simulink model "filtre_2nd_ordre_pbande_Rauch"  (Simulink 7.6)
settings: Solver=ode45  StartTime=0.0  StopTime=10.0  RelTol=1e-3
libraries: fl_lib x8, elec_lib x3, nesl_utility x3

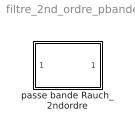
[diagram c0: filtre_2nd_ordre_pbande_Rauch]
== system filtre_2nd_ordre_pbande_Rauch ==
  passe bande Rauch_2ndordre : Subsystem

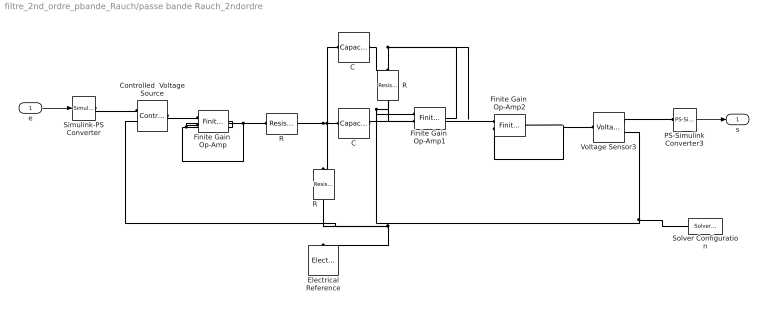
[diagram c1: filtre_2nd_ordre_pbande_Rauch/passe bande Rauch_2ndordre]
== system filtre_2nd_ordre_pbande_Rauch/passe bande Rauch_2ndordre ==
  e : Inport
  C : fl_lib/Electrical/Electrical Elements/Capacitor  DialogController=NetworkEngine.DynNeDlgSource  SystemSampleTime=-1  c=1e-6 F  v0=0 V  r=1e-6 Ohm  g=0 1/Ohm  i_Log=off  v_Log=off  vc_Log=off  LocalVarNames=|i|v|vc  LocalVarDescs=|i|v|Internal variable for voltage across capacitor term  LocalVarLogging=[0 0 0]
  "C " : fl_lib/Electrical/Electrical Elements/Capacitor  DialogController=NetworkEngine.DynNeDlgSource  SystemSampleTime=-1  c=1e-6 F  v0=0 V  r=1e-6 Ohm  g=0 1/Ohm  i_Log=off  v_Log=off  vc_Log=off  LocalVarNames=|i|v|vc  LocalVarDescs=|i|v|Internal variable for voltage across capacitor term  LocalVarLogging=[0 0 0]
  Controlled  Voltage Source : fl_lib/Electrical/Electrical Sources/Controlled Voltage Source  DialogController=NetworkEngine.DynNeDlgSource  SystemSampleTime=-1  i_Log=off  v_Log=off  LocalVarNames=|i|v  LocalVarDescs=|i|v  LocalVarLogging=[0 0]
  Electrical Reference : fl_lib/Electrical/Electrical Elements/Electrical Reference  DialogController=NetworkEngine.DynNeDlgSource  SystemSampleTime=-1  i_Log=off  LocalVarNames=|i  LocalVarDescs=|i  LocalVarLogging=0
  Finite Gain  Op-Amp : elec_lib/Integrated Circuits/Finite Gain Op-Amp  DialogController=NetworkEngine.DynNeDlgSource  SystemSampleTime=-1  A=1000  Rin=1e+6 Ohm  Rout=100 Ohm  Vmin=-15 V  Vmax=15 V  LocalVarLogging=[]
  Finite Gain  Op-Amp1 : elec_lib/Integrated Circuits/Finite Gain Op-Amp  DialogController=NetworkEngine.DynNeDlgSource  SystemSampleTime=-1  A=1000  Rin=1e+6 Ohm  Rout=100 Ohm  Vmin=-15 V  Vmax=15 V  LocalVarLogging=[]
  Finite Gain  Op-Amp2 : elec_lib/Integrated Circuits/Finite Gain Op-Amp  DialogController=NetworkEngine.DynNeDlgSource  SystemSampleTime=-1  A=1000  Rin=1e+6 Ohm  Rout=100 Ohm  Vmin=-15 V  Vmax=15 V  LocalVarLogging=[]
  PS-Simulink Converter3 : nesl_utility/PS-Simulink Converter  DialogController=NetworkEngine.DynNeUtilDlgSource  SystemSampleTime=-1  PhysicalDomain=network_engine_domain  LeftPortType=input  RightPortType=output  SubClassName=ps_output  Unit=1  AffineConversion=off
  R : fl_lib/Electrical/Electrical Elements/Resistor  DialogController=NetworkEngine.DynNeDlgSource  SystemSampleTime=-1  R=1 Ohm  i_Log=off  v_Log=off  LocalVarNames=|i|v  LocalVarDescs=|i|v  LocalVarLogging=[0 0]
  "R " : fl_lib/Electrical/Electrical Elements/Resistor  DialogController=NetworkEngine.DynNeDlgSource  SystemSampleTime=-1  R=1 Ohm  i_Log=off  v_Log=off  LocalVarNames=|i|v  LocalVarDescs=|i|v  LocalVarLogging=[0 0]
  "R   " : fl_lib/Electrical/Electrical Elements/Resistor  DialogController=NetworkEngine.DynNeDlgSource  SystemSampleTime=-1  R=1 Ohm  i_Log=off  v_Log=off  LocalVarNames=|i|v  LocalVarDescs=|i|v  LocalVarLogging=[0 0]
  Simulink-PS Converter : nesl_utility/Simulink-PS Converter  DialogController=NetworkEngine.DynNeUtilDlgSource  SystemSampleTime=-1  PhysicalDomain=network_engine_domain  LeftPortType=input  RightPortType=output  SubClassName=ps_input  Unit=1  AffineConversion=off  InputFilterTimeConstant=.001  UdotUserProvided=0
  Solver Configuration : nesl_utility/Solver Configuration  DialogController=NetworkEngine.DynNeUtilDlgSource  SystemSampleTime=-1  PhysicalDomain=network_engine_domain  LeftPortType=input  RightPortType=generic  SubClassName=solver  Accelerate=off  Profile=off  ResidualTolerance=1e-9  MaxNonlinIter=12  MaxModeIter=2  DoFixedCost=off  UseLocalSampling=off  DoDC=off  LinearAlgebra=Sparse  LocalSolverSampleTime=.001  LocalSolverChoice=NE_BACKWARD_EULER_ADVANCER  UseLocalSolver=off
  Voltage Sensor3 : fl_lib/Electrical/Electrical Sensors/Voltage Sensor  DialogController=NetworkEngine.DynNeDlgSource  SystemSampleTime=-1  i1_Log=off  v1_Log=off  LocalVarNames=|i1|v1  LocalVarDescs=|i1|v1  LocalVarLogging=[]
  s : Outport
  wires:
  PS-Simulink Converter3/1 -> s/1
  e/1 -> Simulink-PS Converter/1
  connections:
  C/LConn1 -- R/RConn1 -- "R "/LConn1 -- "C "/LConn1
  C/RConn1 -- Finite Gain  Op-Amp1/LConn2
  "C "/RConn1 -- "R   "/LConn1 -- Finite Gain  Op-Amp1/RConn1 -- Finite Gain  Op-Amp2/LConn1
  Voltage Sensor3/RConn2 -- "R "/RConn1 -- Electrical Reference/LConn1 -- Controlled  Voltage Source/RConn2 -- Finite Gain  Op-Amp1/LConn1 -- "R   "/RConn1 -- Solver Configuration/RConn1
  Finite Gain  Op-Amp/LConn2 -- Finite Gain  Op-Amp/RConn1 -- R/LConn1
  Finite Gain  Op-Amp2/LConn2 -- Finite Gain  Op-Amp2/RConn1 -- Voltage Sensor3/LConn1
  Simulink-PS Converter/RConn1 -- Controlled  Voltage Source/RConn1
  Controlled  Voltage Source/LConn1 -- Finite Gain  Op-Amp/LConn1
  Voltage Sensor3/RConn1 -- PS-Simulink Converter3/LConn1
